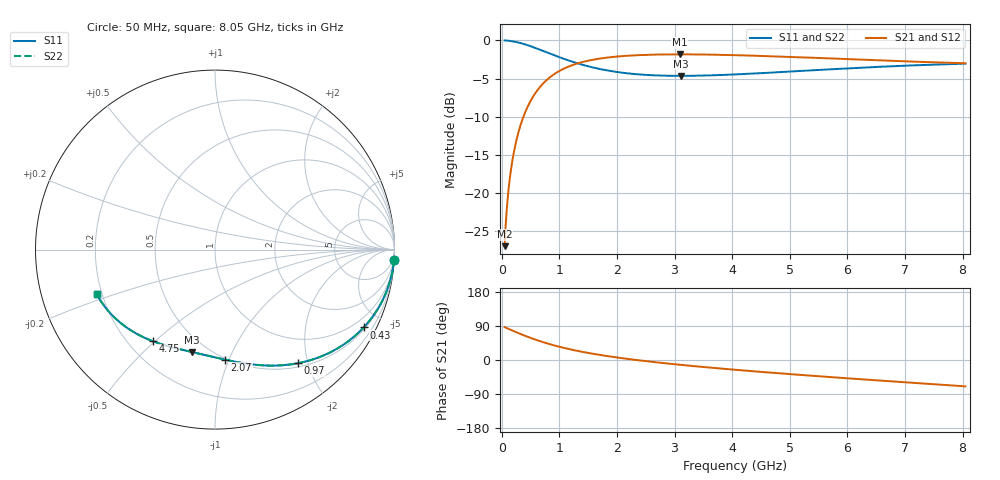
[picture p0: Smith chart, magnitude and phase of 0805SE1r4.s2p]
! AVX Thin Film Operation		Date: August 2001
! Description: Accu-P® Series, Thin Film, SMD, RF Capacitor
! Part Number: 08051J1R4ABT
! 50 MHz  -  8.05 GHz
! Serial Measurements
# mhz S db R 50
!	S11		S21		S12		S22
!	dB	Phase	dB	Phase	dB	Phase	dB	Phase
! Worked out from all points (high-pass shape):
!   401 points, 50 MHz to 8.05 GHz, reference 50 ohm
!   highest |S21| = -1.83 dB at 3.09 GHz (marker M1); lowest = -27.0 dB at 50 MHz (marker M2)
!   |S21| within 3 dB of the highest: 837.9 MHz to end of sweep
!   lowest |S11| = -4.6 dB at 3.11 GHz (marker M3), VSWR 3.82, Z = 20.5 - j35.6 ohm
!   |S11| at or under -10 dB: nowhere
!   |S22| runs from -4.6 to 0.0 dB; largest |S21 - S12| = 0
!   S11 on the Smith chart (normalised r, x): 50 MHz: 1, -34; 430 MHz: 0.58, -3.99; 970 MHz: 0.56, -1.83; 2.07 GHz: 0.49, -0.97; 4.75 GHz: 0.30, -0.49; 8.05 GHz: 0.18, -0.18
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50  -0.01 -3.4  -26.97 86.6  -26.97 86.6  -0.01 -3.4
70  -0.02 -4.7  -24.06 85.3  -24.06 85.3  -0.02 -4.7
130  -0.06 -8.7  -18.73 81.3  -18.73 81.3  -0.06 -8.7
190  -0.12 -12.7  -15.52 77.3  -15.52 77.3  -0.12 -12.7
230  -0.18 -15.3  -13.93 74.7  -13.93 74.7  -0.18 -15.3
290  -0.28 -19.1  -12.05 70.9  -12.05 70.9  -0.28 -19.1
430  -0.58 -27.6  -9.02 62.4  -9.02 62.4  -0.58 -27.6
550  -0.90 -34.4  -7.30 55.6  -7.30 55.6  -0.90 -34.4
670  -1.24 -40.6  -6.06 49.4  -6.06 49.4  -1.24 -40.6
970  -2.12 -53.9  -4.14 36.1  -4.14 36.1  -2.12 -53.9
1170  -2.65 -61.2  -3.40 28.8  -3.40 28.8  -2.65 -61.2
1390  -3.17 -68.2  -2.86 21.8  -2.86 21.8  -3.17 -68.2
1710  -3.76 -76.7  -2.38 13.3  -2.38 13.3  -3.76 -76.7
2070  -4.21 -84.8  -2.07 5.2  -2.07 5.2  -4.21 -84.8
2730  -4.60 -96.8  -1.85 -6.9  -1.85 -6.9  -4.60 -96.8
3090  -4.65 -102.5  -1.83 -12.6  -1.83 -12.6  -4.65 -102.5
3110  -4.65 -102.8  -1.83 -12.9  -1.83 -12.9  -4.65 -102.8
4050  -4.46 -115.7  -1.93 -25.8  -1.93 -25.8  -4.46 -115.7
4750  -4.19 -124.2  -2.09 -34.3  -2.09 -34.3  -4.19 -124.2
5390  -3.92 -131.5  -2.27 -41.6  -2.27 -41.6  -3.92 -131.5
6730  -3.40 -145.9  -2.67 -56.0  -2.67 -56.0  -3.40 -145.9
8050  -3.05 -159.4  -3.00 -69.5  -3.00 -69.5  -3.05 -159.4
